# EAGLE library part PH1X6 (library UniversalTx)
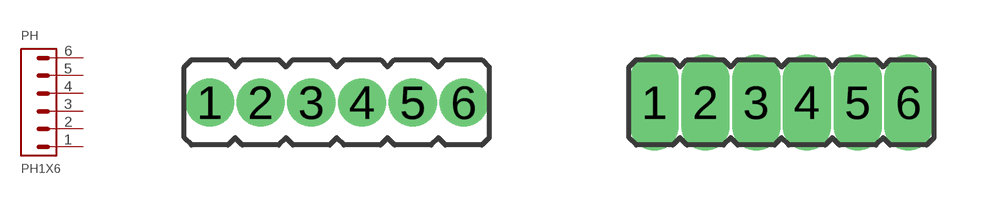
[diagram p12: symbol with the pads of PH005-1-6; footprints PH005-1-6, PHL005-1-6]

Designator prefix PH

## PH1X6-05  [PH005-1-6]
1  1
2  2
3  3
4  4
5  5
6  6

## PH1X6-05LONG  [PHL005-1-6]
Pads as for PH005-1-6

## PH1X6-05LONGSNAP  [PHLS005-1-6]
Pads as for PH005-1-6

## PH1X6-05SNAP  [PHS005-1-6]
Pads as for PH005-1-6

## Footprint PH005-1-6 (pad centres in mm)
Standard 0.05" (1.27mm) pitch pin header.
drill 0.7 pad 1.016: 1 0,0; 2 1.27,0; 3 2.54,0; 4 3.81,0; 5 5.08,0; 6 6.35,0

## Footprint PHL005-1-6 (pad centres in mm)
Standard 0.05" (1.27mm) pitch pin header. Long pads.
drill 0.7 pad 1.016 long: 1 0,0; 2 1.27,0; 3 2.54,0; 4 3.81,0; 5 5.08,0; 6 6.35,0

## Footprint PHLS005-1-6 (pad centres in mm)
Standard 0.05" (1.27mm) pitch pin header. Long pads. Snap. (Pete Lewis offset 3mil)
drill 0.7 pad 1.016 long: 1 0,0.076; 2 1.27,-0.076; 3 2.54,0.076; 4 3.81,-0.076; 5 5.08,0.076; 6 6.35,-0.076

## Footprint PHS005-1-6 (pad centres in mm)
Standard 0.05" (1.27mm) pitch pin header. Snap. (Pete Lewis offset 3mil)
drill 0.7 pad 1.016: 1 0,0.076; 2 1.27,-0.076; 3 2.54,0.076; 4 3.81,-0.076; 5 5.08,0.076; 6 6.35,-0.076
